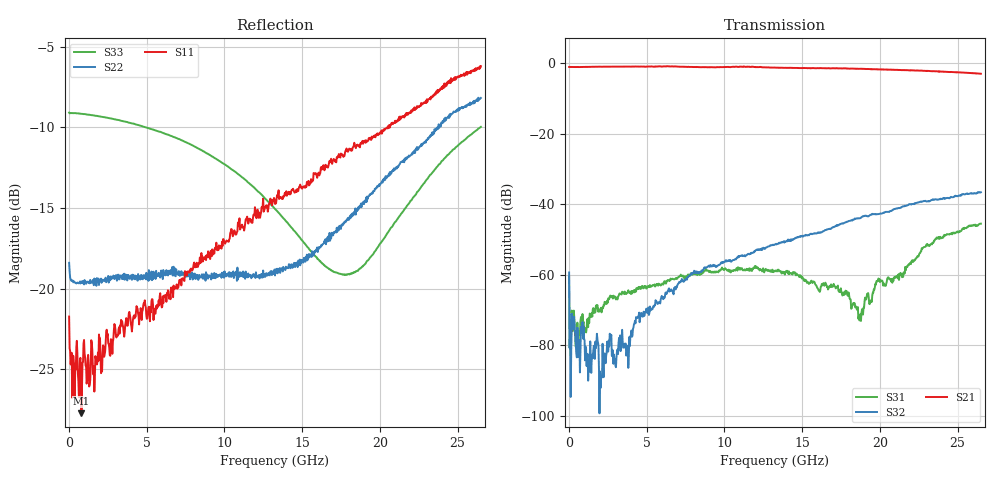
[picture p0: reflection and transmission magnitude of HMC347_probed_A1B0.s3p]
! Hittite Microwave Corporation
! 20 Alpha Road
! Chelmsford, MA 01824
! http://www.hittite.com
! Tel: 978-250-3343
! Fax: 978-250-3373
! Device:  HMC347
! Description: GaAs MMIC SPDT Non-Reflective Switch
! Frequency:  DC -  20.00 GHz
! Package:  DIE
! Ports:  3 RF, 2 DC
!  Pad  1 = RF1 = Port 2
!  Pad  2 = Control A [Alternate]
!  Pad  3 = Control B [Alternate]
!  Pad  4 = RFC = Port 1
!  Pad  5 = Control A [Alternate]
!  Pad  6 = Control B [Alternate]
!  Pad  7 = RF2 = Port 3
!  Pad  8 = Control A
!  Pad  9 = Control B
!  Pad 10 = Control A [Alternate]
! Control:  -5 Volt control voltage
!  Low  = 0 =  0 V
!  High = 1 = -5 V
! State:  RF1 Selected
! Voltages:  VA = -5.0 Volts
!  VB =  0.0 Volts
! Data:  The device was measured using G-S-G Probes at the chip ports.
!  Data was collected using an calibrated 3 port network analyzer.
!  The reference plane is the pads on the switch chip.
! Misc:  Die 64601
!  Lot GB01, Tested Unit 3
! Date Measured:  2010-03-11
! Date:  2010-03-15
! Note:
!  Hittite supplies this data as a sample of measured data at the package pin for
!  for this package product.  Your particular data for this product may vary.
!  Data was taken at 25 degrees C.
!  Hittite reserves the right to change this data at anytime.
!S3P File: Measurements: <S11,S12,S13>,
!  <S21,S22,S23>,
!  <S31,S32,S33>:
# Hz S  dB  R 50
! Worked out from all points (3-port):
!   801 points, 10 MHz to 26.5 GHz, reference 50 ohm
!   strongest paths, dB at 10 MHz, 6.633 GHz, 13.26 GHz, 19.88 GHz, 26.5 GHz:
!     S21: -1.1, -1.0, -1.3, -1.9, -3.1
!     S32: -59.4, -64.5, -51.4, -42.8, -36.6
!     S31: -60.5, -61.2, -59.0, -61.8, -45.5
!   lowest |S11| = -27.8 dB at 804.7 MHz (marker M1), VSWR 1.09, Z = 54.2 + j0.657 ohm
!   |S11| at or under -10 dB: start of sweep to 20.52 GHz; 20.56579 GHz to 20.57758 GHz (11.79 MHz wide, 0.0573 % of centre); 20.63843 GHz to 20.63993 GHz (1.495 MHz wide, 0.00724 % of centre)
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1e7  -21.74 -1.1  -1.06 -0.1  -70.98 -175.5
     -1.14 -0.2  -18.41 -0.8  -69.32 -28.6
     -60.54 96.2  -59.36 15.4  -9.08 179.6
1.755625e8  -23.99 0.2  -1.11 -0.9  -71.08 103.4
            -1.16 -0.9  -19.53 -2.3  -71.41 107.3
            -70.14 107.5  -71.06 108.5  -9.11 178.8
8.047e8  -27.75 8.5  -1.05 -4.5  -72.62 38.9
         -1.17 -4.2  -19.65 -6.6  -75.03 12.2
         -72.40 43.4  -75.62 1.4  -9.15 174.3
3.7186e9  -22.08 -0.2  -1.09 -22.3  -64.93 57.6
          -1.03 -22.0  -19.18 -27.5  -78.56 98.6
          -65.13 56.1  -82.25 74.6  -9.65 155.5
7.923888e9  -18.81 -14.0  -1.15 -47.7  -59.85 56.3
            -1.15 -47.9  -19.00 -56.0  -59.75 72.4
            -60.05 56.3  -59.93 71.5  -11.10 127.4
1.3255e10  -14.74 -30.7  -1.41 -80.6  -59.12 34.5
           -1.32 -80.6  -19.19 -66.5  -51.28 3.0
           -59.05 29.3  -51.42 2.0  -15.06 79.5
1.716228e10  -12.06 -43.7  -1.60 -104.9  -63.25 5.3
             -1.51 -105.9  -16.43 -65.7  -46.30 -38.7
             -63.87 3.9  -46.14 -38.8  -19.00 11.7
1.871856e10  -11.23 -48.3  -1.72 -114.9  -72.19 -100.5
             -1.66 -116.2  -14.86 -66.8  -44.11 -59.7
             -72.18 -104.1  -43.98 -60.2  -18.76 -26.8
1.984439e10  -10.37 -51.9  -1.82 -122.2  -61.43 -167.8
             -1.79 -123.5  -13.62 -69.8  -43.11 -75.7
             -61.69 -164.7  -42.84 -76.6  -17.46 -52.1
2.65e10  -6.19 -74.4  -2.86 -167.6  -45.39 127.8
         -3.07 -169.3  -8.17 -101.8  -37.18 -161.1
         -45.53 127.4  -36.64 -162.3  -9.96 -136.3
